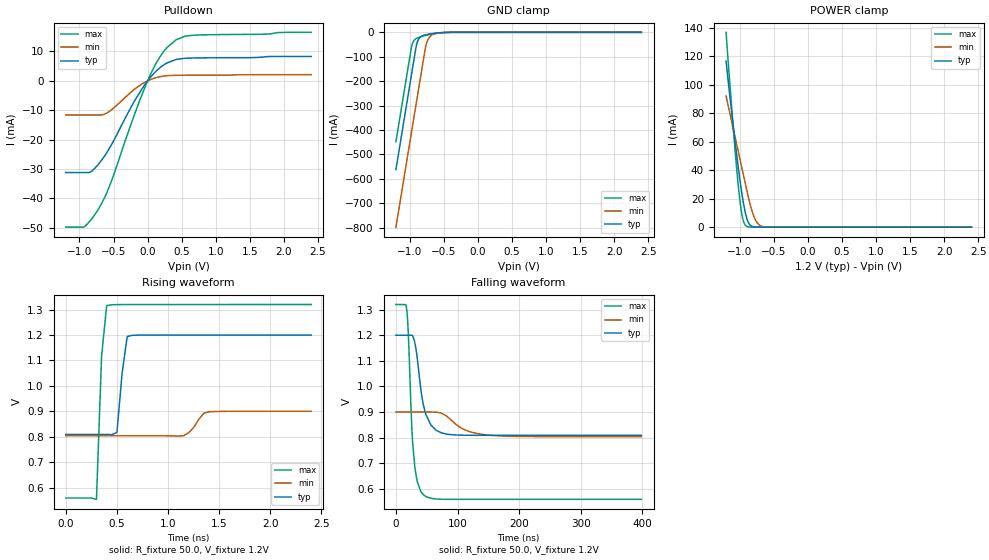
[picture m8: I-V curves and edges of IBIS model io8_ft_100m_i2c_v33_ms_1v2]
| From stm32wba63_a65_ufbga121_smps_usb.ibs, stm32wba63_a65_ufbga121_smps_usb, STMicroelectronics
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[Model]   io8_ft_100m_i2c_v33_ms_1v2
Model_type I/O_open_drain
Polarity   Non-Inverting
Enable   Active-Low
| CAP_THRESHOLD on pad IOFT is "UDTCAPC" :
| Rising=30.0% of vddiom   Falling=70.0% of vddiom
| C_comp min and max val. don't necessarily correlate with the min and max pvt
| but are the smallest and greatest pad capacitance found.
| var   typ   min   max
C_comp   2.85343pF  2.76987pF  2.96512pF
|C_comp_pulldown   2.85343pF  2.76987pF  2.96512pF
Vinl = 450.0mV
Vinh = 660.0mV
Vmeas = 600.0mV   | Reference voltage for timing measurements
Cref  = 50.0pF   | Timing specification test load capacitance value
Rref  = 1.0MOhm   | Timing specification test load resistance value
Vref  = 660.0mV   | Timing specification test load voltage
[Model Spec]
| TIME_THRESHOLD on pin ZII2CV11 is "CMOS" :
| Rising=50.0% of vdd   Falling=50.0% of vdd
Vinl 436.50000mV 331.50000mV 482.50000mV
Vinh 753.50000mV 549.50000mV 837.50000mV
| variable   typ   min   max
[Temperature Range] 25.0 140.0 -40.0
| variable   typ   min   max
[Voltage Range] 1.2V 900.0mV 1.32V
| variable   typ   min   max
[POWER Clamp Reference] 1.2V 900.0mV 1.32V
| variable   typ   min   max
[GND Clamp Reference] 0V 0V 0V
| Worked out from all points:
|   slope of the pulldown table from 0 to 0.18 V, typ, clamps not added: 40.6 ohm
|   GND clamp passes 1 mA (typ) near -0.51 V on its own axis
|   POWER clamp passes 1 mA (typ) near -0.83 V on its own axis
|   rising waveform, R_fixture 50.0, V_fixture 1.2V: 20-80 % time 60.1ps typ, 108ps min, 48.7ps max; typ from 0.809 V to 1.2 V
|   falling waveform, R_fixture 50.0, V_fixture 1.2V: 20-80 % time 15.3ns typ, 36.5ns min, 8.91ns max; typ from 1.2 V to 0.809 V
[POWER Clamp]
-1.2V     116.7mA    92.13mA    136.9mA
-1.09V    69.42mA    68.21mA    67.14mA
-1.02V    41.75mA    52.99mA    28.91mA
-990mV    30.98mA    46.47mA    16.09mA
-970mV    24.36mA    42.12mA    9.575mA
-940mV    15.59mA    35.6mA     3.485mA
-910mV    8.693mA    29.07mA    1.01mA
-860mV    2.259mA    18.59mA    104.6uA
-780mV    143.1uA    6.246mA    2.555uA
-720mV    16.22uA    1.846mA    157.1nA
-650mV    1.267uA    330.3uA    6.118nA
2.4V      0A         0A         0A
[GND Clamp]
-1.2V     -561.6mA   -797.4mA   -447.4mA
-980mV    -187.6mA   -423.4mA   -73.43mA
-960mV    -153.6mA   -389.4mA   -48.26mA
-900mV    -54.17mA   -287.4mA   -24.97mA
-870mV    -29.55mA   -236.4mA   -21.19mA
-830mV    -17.05mA   -168.4mA   -17.42mA
-760mV    -9.921mA   -54.55mA   -11.89mA
-730mV    -8.191mA   -29.78mA   -9.811mA
-690mV    -6.26mA    -14.49mA   -7.318mA
-600mV    -2.976mA   -4.315mA   -3.058mA
-380mV    -57.63uA   -251uA     -19.49uA
2.4V      872.8pA    204.8nA    349.4pA
| variable   typ   min   max
[Pullup Reference] 1.2V 900.0mV 1.32V
| variable   typ   min   max
[Pulldown Reference] 0V 0V 0V
[Pulldown]
-1.2V     -31.2mA    -11.62mA   -49.78mA
-930mV    -31.2mA    -11.62mA   -49.64mA
-830mV    -30.86mA   -11.62mA   -47.25mA
-710mV    -28.04mA   -11.62mA   -43.19mA
-550mV    -22.55mA   -10.2mA    -35.3mA
-200mV    -7.146mA   -2.964mA   -11.89mA
40mV      1.171mA    405.8uA    2.092mA
130mV     3.416mA    1.118mA    6.182mA
230mV     5.302mA    1.613mA    9.763mA
420mV     7.288mA    1.898mA    13.99mA
670mV     7.779mA    1.924mA    15.51mA
2.4V      8.312mA    2.101mA    16.51mA
[Ramp]
dV/dt_r 234.64854mV/734.3138ps 57.85916mV/2.01414ns 456.7237mV/408.59668ps
dV/dt_f 234.6598mV/15.09514ns 57.89516mV/35.99396ns 456.73592mV/8.71403ns
R_load = 50.0
| Removed startup time: 0s 0s 0s  .
| Removed end time: 2.4ns.
[Rising Waveform]
R_fixture   = 50.0
V_fixture   = 1.2V
V_fixture_min = 900.0mV
V_fixture_max = 1.32V
0s        808.9mV    803.5mV    558.8mV
300ps     808.9mV    803.5mV    553.5mV
350ps     808.9mV    803.5mV    1.118V
400ps     808.9mV    803.5mV    1.316V
500ps     816.3mV    803.5mV    1.319V
550ps     1.047V     803.5mV    1.32V
600ps     1.194V     803.5mV    1.32V
1.15ns    1.2V       803.7mV    1.32V
1.4ns     1.2V       897.7mV    1.32V
2.4ns     1.2V       899.9mV    1.32V
| Removed startup time: 0s 0s 0s  .
| Removed end time: 398.4ns.
[Falling Waveform]
R_fixture   = 50.0
V_fixture   = 1.2V
V_fixture_min = 900.0mV
V_fixture_max = 1.32V
0s        1.2V       900mV      1.32V
17.2ns    1.2V       900mV      1.305V
20ns      1.2V       900mV      1.212V
26.15ns   1.2V       900mV      823.1mV
30.4ns    1.175V     900mV      691.3mV
46.7ns    906.7mV    900mV      572.7mV
65.05ns   829mV      899.7mV    560.2mV
86.4ns    812.4mV    875.9mV    558.9mV
146.4ns   808.9mV    810.8mV    558.8mV
398.4ns   808.9mV    803.5mV    558.8mV
